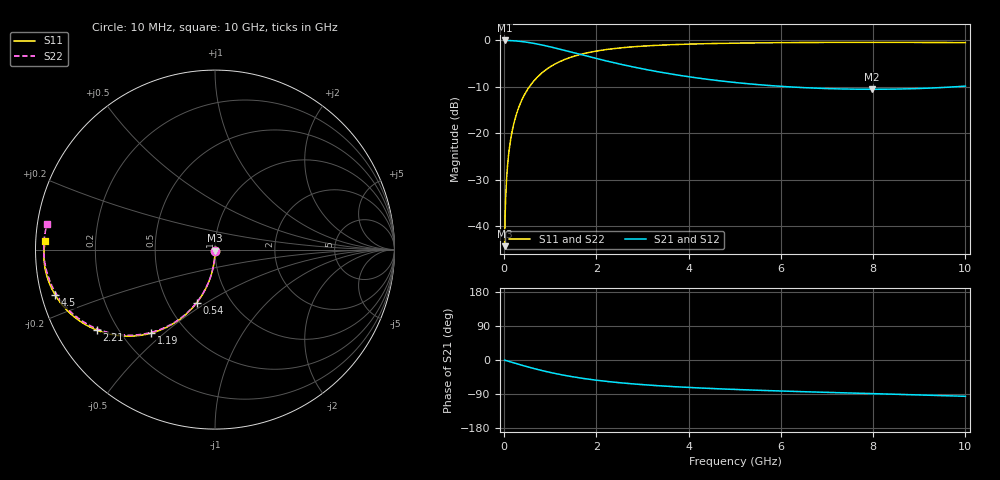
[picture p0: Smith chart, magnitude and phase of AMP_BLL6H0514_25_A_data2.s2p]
! Created Wed Apr 14 10:48:13 2010
# ghz S ma R 50
! 2 Port Network Data from SP1.SP block
! freq  magS11  angS11  magS21  angS21  magS12  angS12  magS22  angS22
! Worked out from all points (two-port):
!   1000 points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, 10 MHz to 10 GHz, reference 50 ohm
!   highest |S21| = 0.00 dB at 10 MHz (marker M1); lowest = -10.5 dB at 7.98 GHz (marker M2)
!   |S21| within 3 dB of the highest: start of sweep to 1.648 GHz
!   lowest |S11| = -44.3 dB at 10 MHz (marker M3), VSWR 1.01, Z = 50 - j0.613 ohm
!   |S11| at or under -10 dB: start of sweep to 544.5 MHz
!   |S22| runs from -44.3 to -0.4 dB; largest |S21 - S12| = 0
!   S11 on the Smith chart (normalised r, x): 10 MHz: 1.00, -0.01; 540 MHz: 0.69, -0.46; 1.19 GHz: 0.32, -0.45; 2.21 GHz: 0.12, -0.30; 4.5 GHz: 0.04, -0.14; 10 GHz: 0.03, +0.02
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0.01  0.006128 -90.4  1 -0.4  1 -0.4  0.006128 -90.4
0.03  0.01838 -91.1  0.9998 -1.1  0.9998 -1.1  0.01838 -91.1
0.07  0.04286 -92.5  0.9991 -2.6  0.9991 -2.6  0.04286 -92.6
0.08  0.04896 -92.9  0.9988 -2.9  0.9988 -2.9  0.04896 -92.9
0.11  0.06725 -94.0  0.9977 -4.0  0.9977 -4.0  0.06725 -94.0
0.16  0.09757 -95.8  0.9952 -5.8  0.9952 -5.8  0.09757 -95.9
0.23  0.1395 -98.3  0.9902 -8.4  0.9902 -8.4  0.1395 -98.4
0.31  0.1866 -101.1  0.9824 -11.2  0.9824 -11.2  0.1866 -101.3
0.41  0.2436 -104.6  0.9699 -14.7  0.9699 -14.7  0.2436 -104.8
0.54  0.3139 -109.0  0.9494 -19.1  0.9494 -19.1  0.3139 -109.2
0.82  0.4481 -117.7  0.894 -27.8  0.894 -27.8  0.4481 -118.0
1.19  0.587 -127.5  0.8096 -37.7  0.8096 -37.7  0.587 -128.0
1.68  0.7128 -137.7  0.7013 -48.0  0.7013 -48.0  0.7128 -138.4
2.21  0.7977 -145.8  0.6031 -56.3  0.6031 -56.3  0.7977 -146.8
2.73  0.8496 -151.8  0.5274 -62.4  0.5274 -62.4  0.8496 -153.0
3.34  0.8877 -157.1  0.4603 -67.9  0.4603 -67.9  0.8877 -158.6
4.5  0.9262 -164.2  0.377 -75.3  0.377 -75.3  0.9262 -166.3
5.01  0.9356 -166.6  0.3529 -77.8  0.3529 -77.8  0.9356 -168.9
6.67  0.9513 -172.7  0.308 -84.3  0.308 -84.3  0.9513 -175.9
7.98  0.9544 -176.6  0.2984 -88.7  0.2984 -88.7  0.9544 179.2
8.34  0.9542 -177.7  0.2991 -89.9  0.2991 -89.9  0.9541 177.9
10  0.9464 177.2  0.3228 -95.8  0.3228 -95.8  0.9463 171.2
